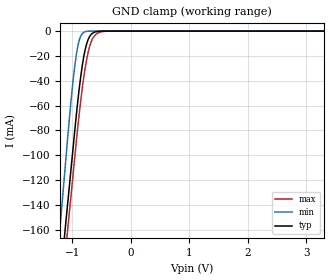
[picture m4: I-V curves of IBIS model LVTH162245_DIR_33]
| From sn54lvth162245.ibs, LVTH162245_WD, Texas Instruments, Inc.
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[Model]   LVTH162245_DIR_33
Model_type  Input
Vinl = 0.8
Vinh = 2.0
| variable   typ   min   max
C_comp   3.55pF   2.62pF   4.44pF
[Temperature Range]   40   -40   100
| Ambient temperature   25   -40   85
[Voltage range]   3.3   3   3.6
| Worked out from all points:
|   GND clamp passes 1 mA (typ) near -0.62 V on its own axis
[GND Clamp]
| LVTH162245_DIR_33
|   Voltage   I(typ)   I(min)   I(max)
-5.5V     -2.288A    -2.547A    -2.284A
-1.225V   -210.8mA   -168.1mA   -231.1mA
-1.195V   -196.3mA   -151.5mA   -216.7mA
-1.135V   -167.2mA   -118.2mA   -187.9mA
-1.105V   -152.7mA   -101.6mA   -173.6mA
-1.075V   -138.1mA   -84.99mA   -159.2mA
-975mV    -89.73mA   -35.97mA   -111.2mA
-900mV    -54.95mA   -11.36mA   -75.86mA
-775mV    -14.49mA   -458.2uA   -29.04mA
-700mV    -4.229mA   -21.87uA   -12.08mA
-600mV    -595.8uA   -186.1nA   -2.835mA
3.3V      11.11pA    3.42pA     1.265nA
